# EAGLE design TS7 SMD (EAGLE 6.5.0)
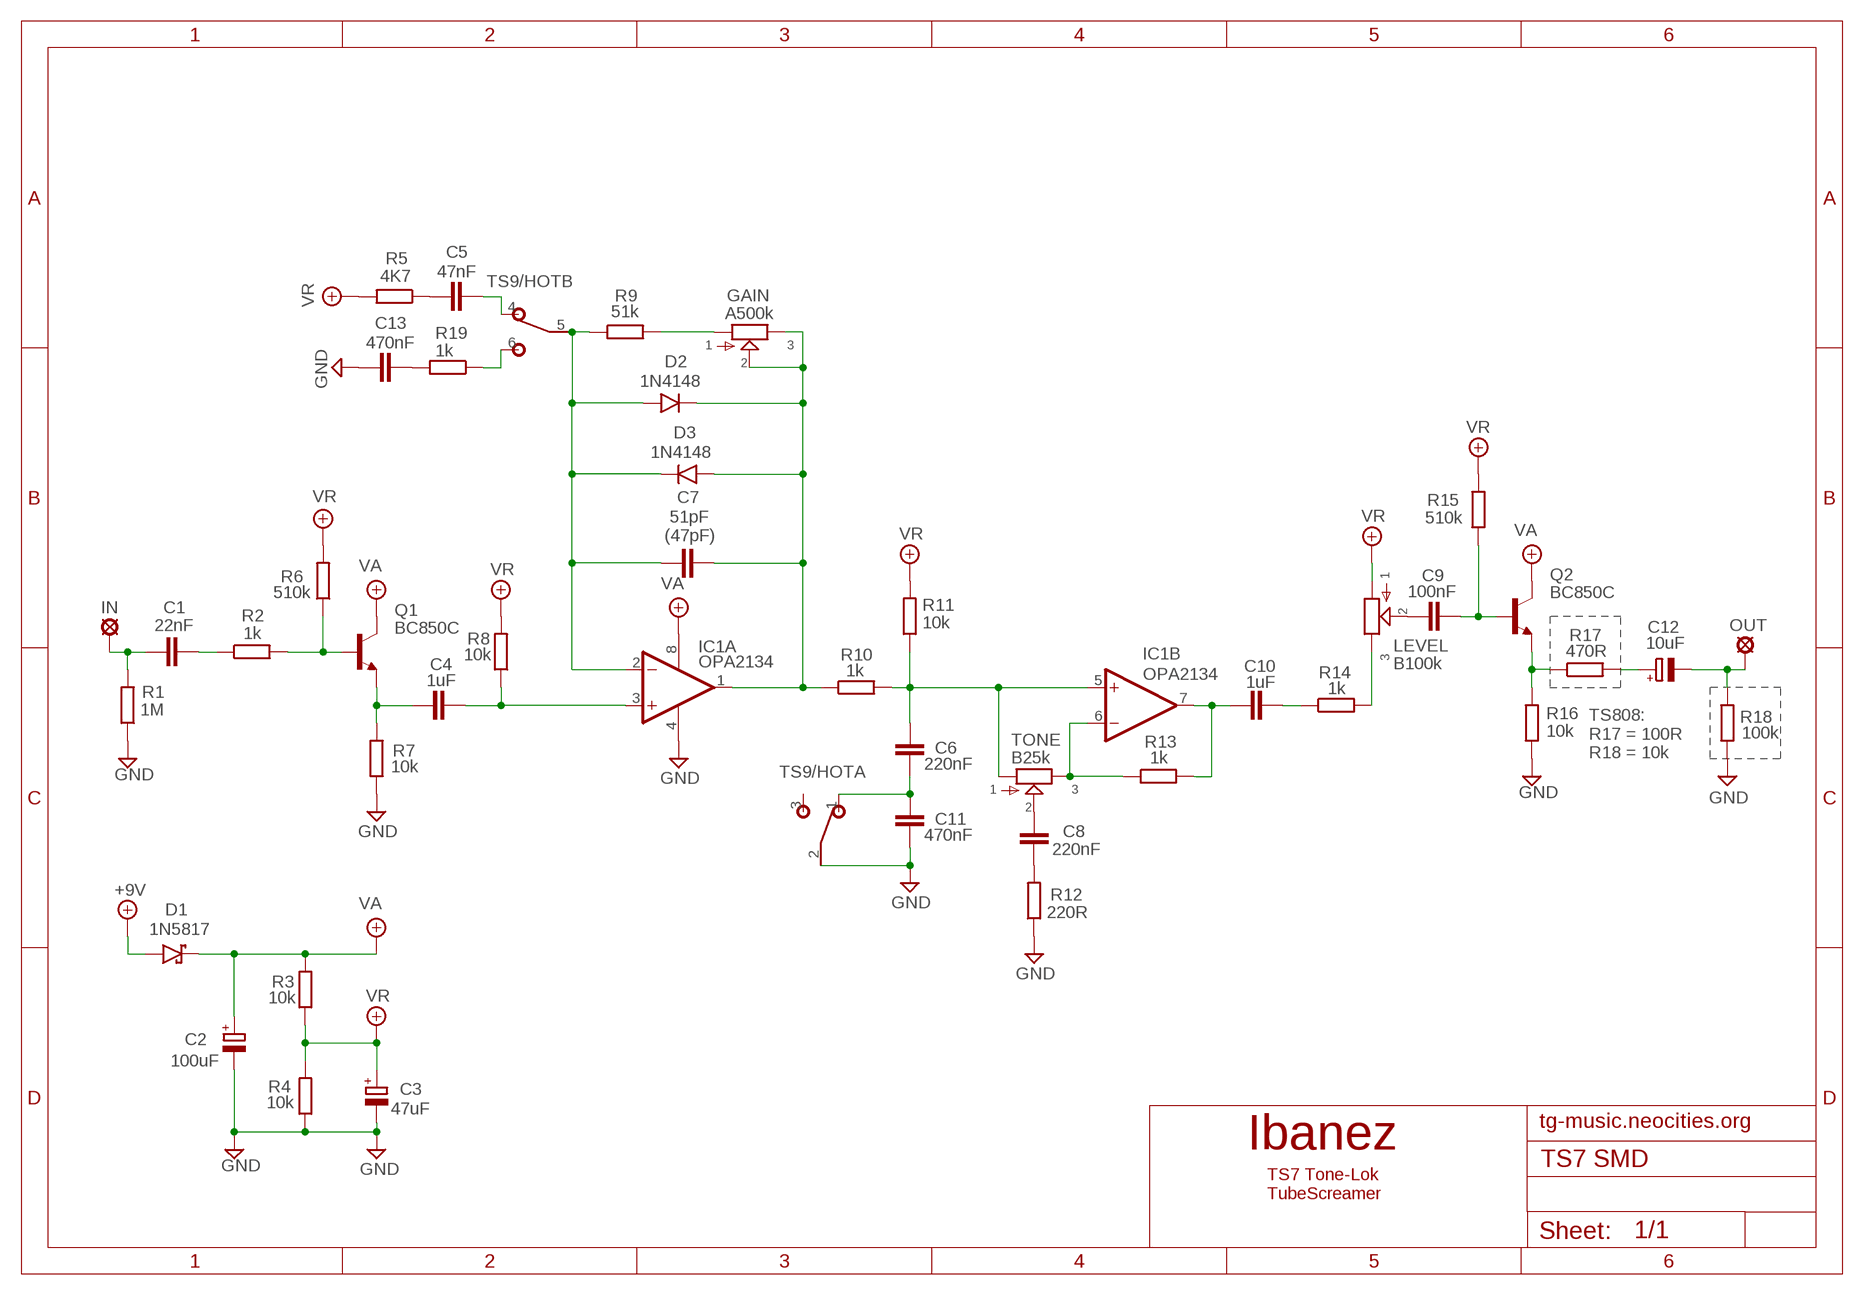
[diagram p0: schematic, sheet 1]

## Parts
+9V  +9V  +9V(T)1  [ROUND]
C1  22nF  C-EUC0805  [C0805]
C2  100uF  CPOL-EUD  [PANASONIC_D]
C3  47uF  CPOL-EUC  [PANASONIC_C]
C4  1uF  C-EUC0805  [C0805]
C5  47nF  C-EUC0805  [C0805]
C6  220nF  C-EUC0805  [C0805]
C7  51pF  C-EUC0805  [C0805]
C8  220nF  C-EUC0805  [C0805]
C9  100nF  C-EUC0805  [C0805]
C10  1uF  C-EUC0805  [C0805]
C11  470nF  C-EUC0805  [C0805]
C12  10uF  CPOL-EUB  [PANASONIC_B]
C13  470nF  C-EUC0805  [C0805]
D1  1N5817  1N5817SMD  [MELF-MLL41_DO213AB]
D2  1N4148  1N4148SMD  [SOD123]
D3  1N4148  1N4148SMD  [SOD123]
GAIN  A500k  POT-EU9MM  [9MM_SNAP-IN_POT]
GND  GND  GND(T)1  [ROUND]
GND1  GND  GND(T)1  [ROUND]
IC1  OPA2134  LM4558D  [SO08]
IN  MCS10B  [MCS10B]
LEVEL  B100k  POT-EU9MM  [9MM_SNAP-IN_POT]
OUT  MCS10B  [MCS10B]
Q1  BC850C  BC847ALT1SMD  [SOT23]
Q2  BC850C  BC847ALT1SMD  [SOT23]
R1  1M  R-EU_R0805  [R0805]
R2  1k  R-EU_R0805  [R0805]
R3  10k  R-EU_R0805  [R0805]
R4  10k  R-EU_R0805  [R0805]
R5  4K7  R-EU_R0805  [R0805]
R6  510k  R-EU_R0805  [R0805]
R7  10k  R-EU_R0805  [R0805]
R8  10k  R-EU_R0805  [R0805]
R9  51k  R-EU_R0805  [R0805]
R10  1k  R-EU_R0805  [R0805]
R11  10k  R-EU_R0805  [R0805]
R12  220R  R-EU_R0805  [R0805]
R13  1k  R-EU_R0805  [R0805]
R14  1k  R-EU_R0805  [R0805]
R15  510k  R-EU_R0805  [R0805]
R16  10k  R-EU_R0805  [R0805]
R17  470R  R-EU_R0805  [R0805]
R18  100k  R-EU_R0805  [R0805]
R19  1k  R-EU_R0805  [R0805]
TONE  B25k  POT-EU9MM  [9MM_SNAP-IN_POT]
TS9/HOT  DPDTTHT  [M9040P2]

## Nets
+9V: +9V.1(+9V) D1.A
GND: C2.- C3.- C11.2 C13.1 GND1.1(GND) GND.1(GND) IC1.4(P:V-) R1.1 R4.1 R7.1 R12.1 R16.1 R18.1 TS9/HOT.2
N$1: C8.1 TONE.2
N$2: C1.2 R2.1
N$3: Q1.1(B) R2.2 R6.1
N$4: C4.2 IC1.3(A:+IN) R8.1
N$5: C7.1 D2.A D3.C IC1.2(A:-IN) R9.1 TS9/HOT.5
N$6: C4.1 Q1.2(E) R7.2
N$7: C8.2 R12.2
N$8: GAIN.1 R9.2
N$9: C9.1 LEVEL.2
N$10: IC1.6(B:-IN) R13.1 TONE.3
N$11: C6.1 IC1.5(B:+IN) R10.2 R11.1 TONE.1
N$12: C6.2 C11.1 TS9/HOT.1
N$13: C7.2 D2.C D3.A GAIN.2 GAIN.3 IC1.1(A:OUT) R10.1
N$15: C10.2 R14.1
N$16: LEVEL.3 R14.2
N$17: Q2.2(E) R16.2 R17.1
N$18: C1.1 IN.MP R1.2
N$19: C9.2 Q2.1(B) R15.1
N$20: C12.+ R17.2
N$21: C12.- OUT.MP R18.2
N$22: C13.2 R19.2
N$23: C5.1 R5.1
N$24: C5.2 TS9/HOT.4
N$25: R19.1 TS9/HOT.6
N$26: C10.1 IC1.7(B:OUT) R13.2
VA: C2.+ D1.C IC1.8(P:V+) Q1.3(C) Q2.3(C) R3.2
VR: C3.+ LEVEL.1 R3.1 R4.2 R5.2 R6.2 R8.2 R11.2 R15.2
Unconnected: TS9/HOT.3

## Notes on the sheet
- (47pF)
- TS808:
  R17 = 100R
  R18 = 10k
- tg-music.neocities.org
- Ibanez
- TS7 Tone-Lok
  TubeScreamer

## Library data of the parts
+9V = gm-supply:+9V(T): +9V Voltage Supply
C1 C4-C11 C13 = rcl:C-EU: CAPACITOR, European symbol
C2 C3 C12 = rcl:CPOL-EU: POLARIZED CAPACITOR, European symbol
D1 = Diodit:1N5817
D2 D3 = Diodit:1N4148: Fast Switching Diode
GAIN LEVEL TONE = potentiometers:POT-EU
GND GND1 = gm-supply:GND(T): Ground
IC1 = Operaatiovahvistimet:*4558: *4558 Op Amp Infamous for its use in tube screamers. This op amp has many manufacturers, hence the leading "*" in the name. The JRC4558 is a widely used example.
IN OUT = Padit:MCS10B: SOLDER PAD
Q1 Q2 = Transistorit:BC847*: NPN Transistor
R1-R19 = rcl:R-EU_: RESISTOR, European symbol
TS9/HOT = Kytkimet:DPDT

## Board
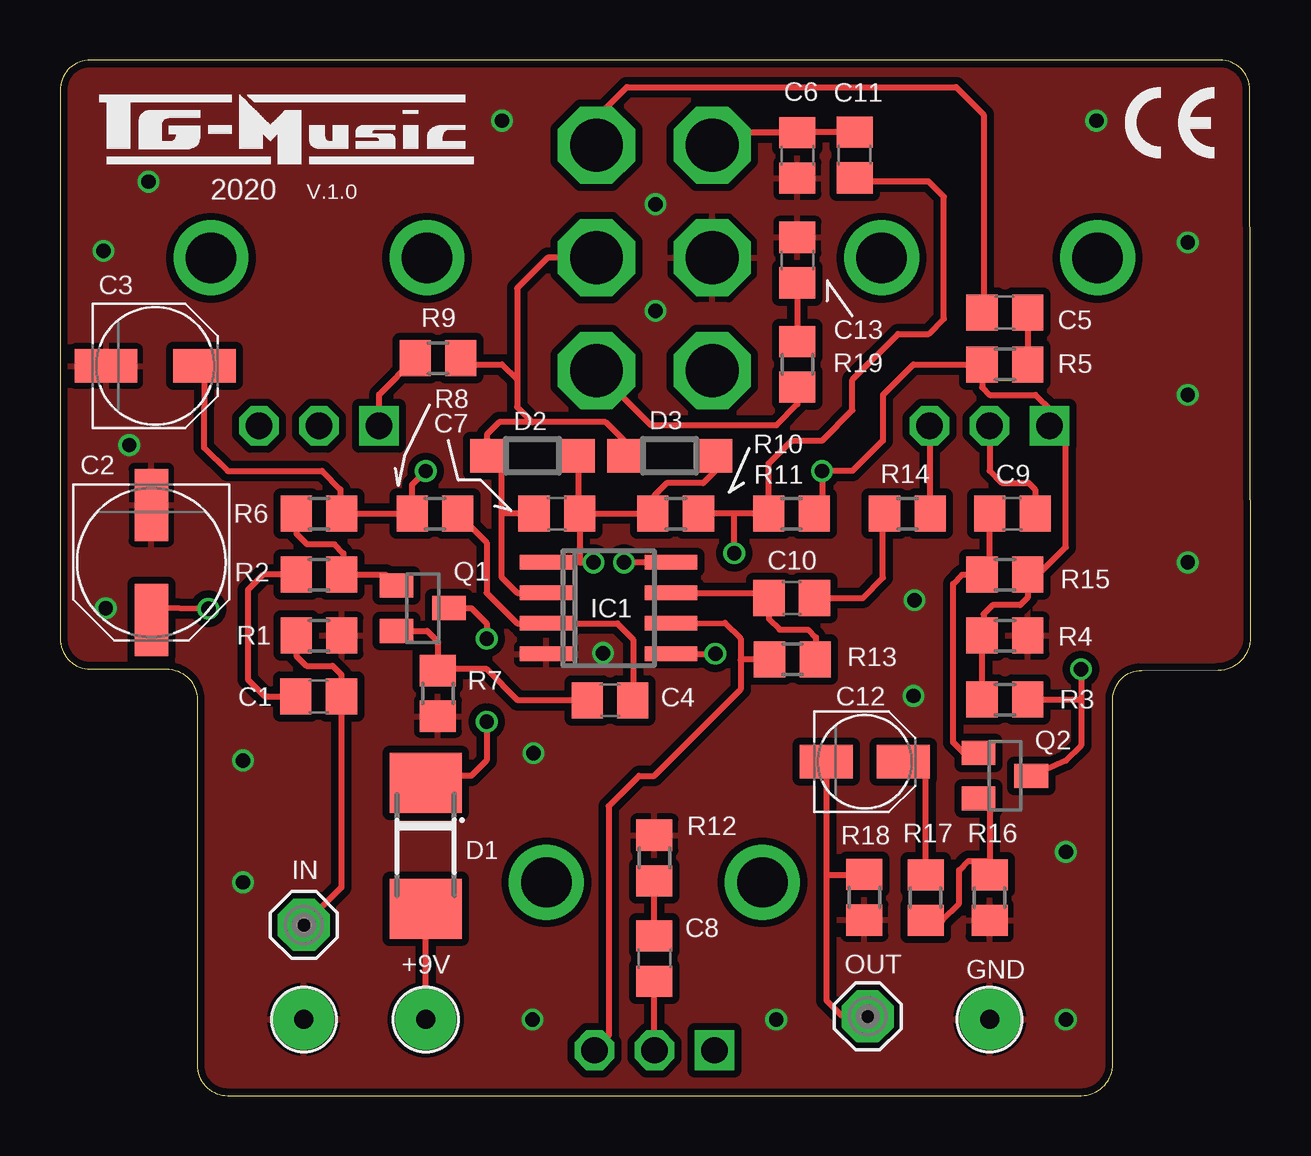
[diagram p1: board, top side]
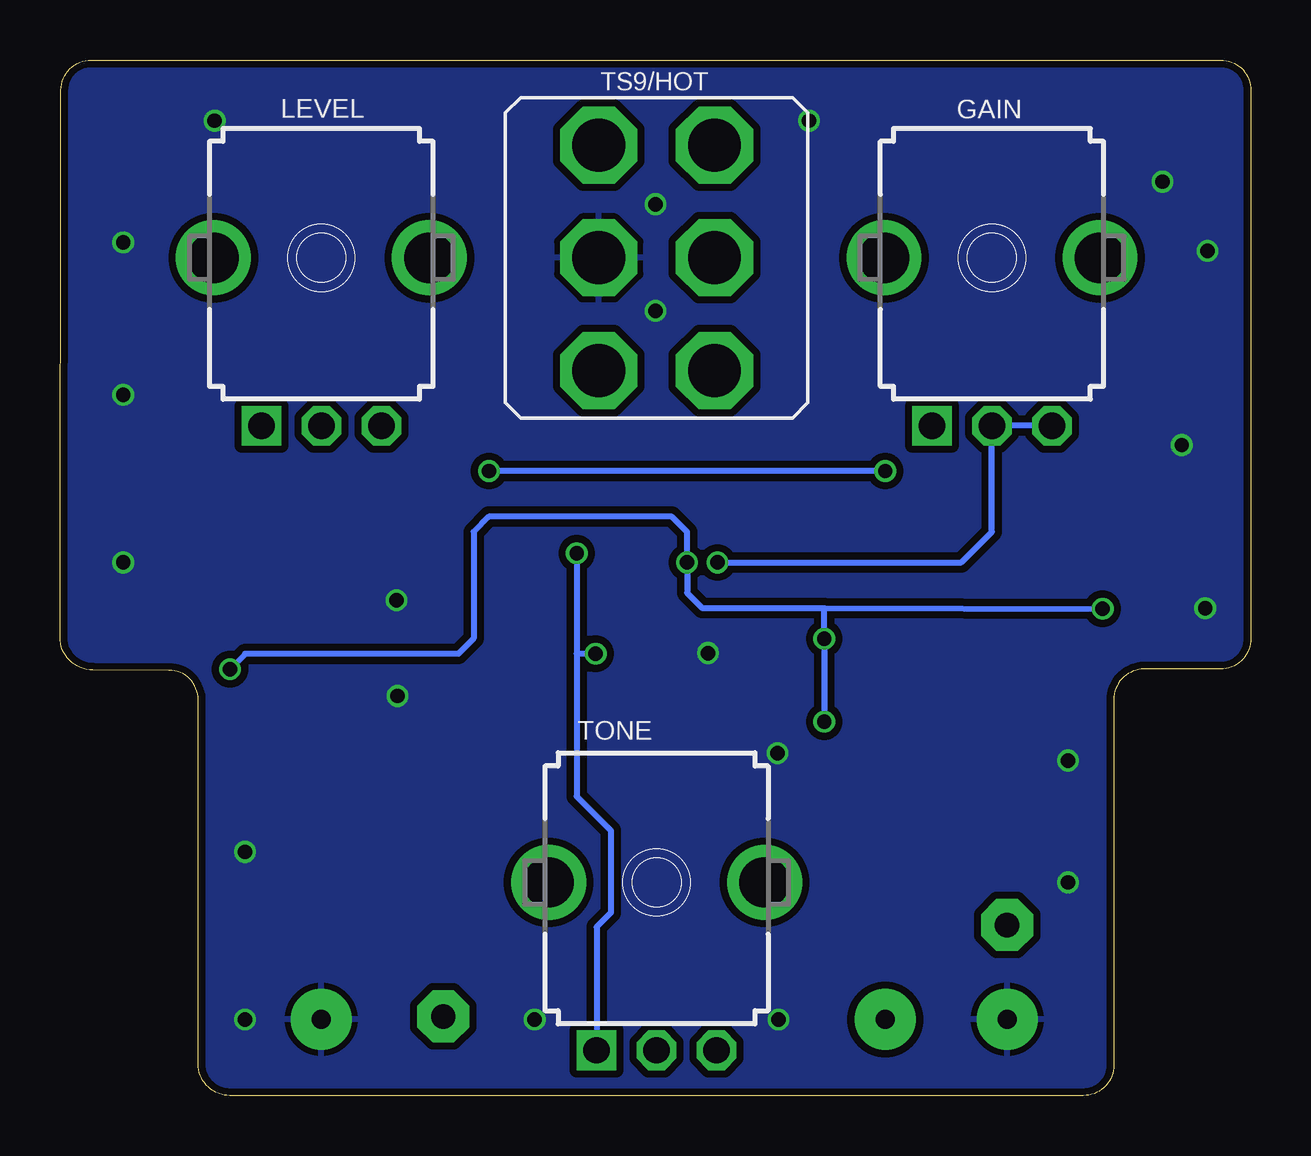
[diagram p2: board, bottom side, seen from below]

Size 49.62 x 43.17 mm. Coordinates in mm from the lower left corner, seen from the top.
Outline: 5.71,16.51 5.71,1.27 arc90 6.99,0 42.55,0 arc90 43.87,1.32 43.87,16.51 arc-90 45.08,17.73 48.26,17.74 arc90 49.62,19.11 49.58,41.91 arc90 48.32,43.17 1.27,43.17 arc90 0,41.9 0,19.05 arc90 1.27,17.78 4.45,17.78 arc-90 5.71,16.51
Copper layers (1*16): Top 0.035mm / dielectric 1.5mm / Bottom 0.035mm
Design rules "ITEADstudio": minimum track width 10mil, minimum drill 12mil, track to track 12mil, track to pad 12mil, pad to pad 12mil, via to via 12mil, smd to smd 0mil, copper to edge 12mil, drill to drill 12mil, minimum pad ring 10mil, minimum via ring 6mil, stop-mask expansion 4mil, vias tented up to drill 100mil, thermal gap 10mil

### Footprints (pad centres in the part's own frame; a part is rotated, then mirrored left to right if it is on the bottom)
ROUND = drill 0.8 pad 2.54: 1 0,0
C0805 = smd 1.3 x 1.5: 1 -0.95,0; 2 0.95,0
PANASONIC_D = smd 3 x 1.4: + 2.4,0; - -2.4,0
PANASONIC_C = smd 2.6 x 1.4: + 2.05,0; - -2.05,0
PANASONIC_B = smd 2.2 x 1.4: + 1.6,0; - -1.6,0
MELF-MLL41_DO213AB = smd 2.5 x 3: A 2.625,0; C -2.625,0
SOD123 = smd 1.4 x 1.4: A 1.9,0; C -1.9,0
9MM_SNAP-IN_POT = drill 1.1 square: 1 -2.5,-7 | drill 1.1 octagon: 2 0,-7; 3 2.5,-7 | drill 2.1 pad 2.794: CHASSIS1 -4.5,0; CHASSIS2 4.5,0
SO08 = smd 0.6 x 2.2: 1 -1.905,-2.6; 2 -0.635,-2.6; 3 0.635,-2.6; 4 1.905,-2.6; 5 1.905,2.6; 6 0.635,2.6; 7 -0.635,2.6; 8 -1.905,2.6
MCS10B = drill 1.016 pad 2.159 octagon: MP 0,0
SOT23 = smd 1 x 1.4: 1 -0.95,-1.1; 2 0.95,-1.1; 3 0,1.1
R0805 = smd 1.3 x 1.5: 1 -0.95,0; 2 0.95,0
M9040P2 = drill 2.2 octagon: 1 -2.413,4.699; 2 -2.413,0; 3 -2.413,-4.699; 4 2.413,4.699; 5 2.413,0; 6 2.413,-4.699

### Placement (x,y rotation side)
+9V  15.24,3.17 0 top
C1  10.78,16.64 180 top
C2  3.81,22.23 270 top
C3  3.97,30.42 0 top
C4  22.92,16.48 0 top
C5  39.37,32.64 180 top
C6  33.11,39.21 90 top
C7  20.7,24.26 0 top
C8  24.77,5.71 90 top
C9  39.68,24.26 180 top
C10  30.49,20.74 0 top
C11  30.72,39.19 270 top
C12  33.53,13.92 0 top
C13  30.72,34.83 270 top
D1  15.24,10.41 270 top
D2  19.68,26.67 180 top
D3  25.4,26.67 0 top
GAIN  10.79,34.92 0 bottom
GND  38.73,3.17 0 top
GND1  10.16,3.17 0 top
IC1  22.86,20.32 270 top
IN  10.16,7.11 0 top
LEVEL  38.73,34.92 0 bottom
OUT  33.66,3.3 0 top
Q1  15.11,20.32 270 top
Q2  39.37,13.34 270 top
R1  10.79,19.18 180 top
R2  10.79,21.72 0 top
R3  39.37,16.51 0 top
R4  39.37,19.18 180 top
R5  39.37,30.48 180 top
R6  10.79,24.26 0 top
R7  15.75,16.76 90 top
R8  15.62,24.26 180 top
R9  15.75,30.73 180 top
R10  25.65,24.26 0 top
R11  30.48,24.26 0 top
R12  24.77,9.91 270 top
R13  30.52,18.19 0 top
R14  35.31,24.26 0 top
R15  39.37,21.72 0 top
R16  38.73,8.26 90 top
R17  36.07,8.26 90 top
R18  33.52,8.27 90 top
R19  30.73,30.48 90 top
TONE  24.77,8.89 0 bottom
TS9/HOT  24.77,34.92 0 bottom

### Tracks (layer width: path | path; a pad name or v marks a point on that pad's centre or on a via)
+9V
  Top 0.254: +9V.1 D1.A
GND  (via drill 0.6)
  other vias: 3.68,38.1 18.41,40.64 43.18,40.64 46.99,35.56 46.99,29.21 46.99,22.23 41.91,10.16 41.91,3.17 29.84,3.17 19.68,3.17 35.56,16.66 7.62,8.89 7.62,13.97 22.63,18.45 19.72,14.28 35.61,20.65 24.81,32.71 24.81,37.16 1.81,35.21 2.88,27.12 1.91,20.32
  pour Top: 5.71,1.27 5.71,16.51 arc90 4.45,17.78 1.27,17.78 arc-90 0,19.05 0,41.91 arc-90 1.27,43.18 48.26,43.18 arc-90 49.53,41.91 49.53,19.05 arc-90 48.26,17.78 45.09,17.78 arc90 43.81,16.51 43.81,1.27 arc-90 42.55,0 6.99,0 arc-90
  pour Bottom: 5.71,1.27 5.71,16.51 arc90 4.45,17.78 1.27,17.78 arc-90 0,19.05 0,41.91 arc-90 1.27,43.18 48.26,43.18 arc-90 49.53,41.91 49.53,19.05 arc-90 48.26,17.78 45.09,17.78 arc90 43.81,16.51 43.81,1.27 arc-90 42.55,0 6.99,0 arc-90
N$1
  Top 0.254: TONE.2 C8.1
N$2
  Top 0.254: R2.1 8.46,21.72 7.83,21.08 7.83,17.35 8.54,16.64 C1.2 | C1.2
N$3
  Top 0.254: Q1.1 13.57,21.72 R2.2 11.81,21.78 11.81,22.61 11.43,22.99 10.29,22.99 9.85,23.43 R6.1
N$4
  Top 0.254: R8.1 17.78,23.05 17.78,20.95 19.05,19.68 IC1.3 23.22,19.68 23.88,19.01 23.88,16.82 C4.2
N$5
  Top 0.254: IC1.2 19.05,20.95 18.41,21.59 18.41,24.26 | D2.A 17.79,26.22 | D2.A 17.79,26.68 | D3.C 23.5,27.3 22.73,28.07 19.68,28.07 | 19.68,28.07 18.29,28.07 17.79,27.56 D2.A | 19.05,29.84 19.05,33.66 20.32,34.92 TS9/HOT.5 | 19.05,29.84 19.05,28.7 19.68,28.07 | R9.1 16.95,30.48 18.41,30.48 19.05,29.84 | 18.41,24.26 18.41,26.04 D2.A | C7.1 18.41,24.26
N$6
  Top 0.254: Q1.2 15.3,19.37 15.75,18.92 R7.2 15.81,17.78 17.78,17.78 19.08,16.48 C4.1
N$7
  Top 0.254: C8.2 R12.2
N$8
  Top 0.254: GAIN.1 13.29,29.23 R9.2
N$9
  Top 0.254: LEVEL.2 38.73,26.05 39.24,25.54 40.35,25.54 40.63,25.27 C9.1
N$10
  Top 0.254: TONE.3 22.86,2.48 22.86,12.06 24.13,13.34 24.77,13.34 28.36,16.93 28.36,18.16 | IC1.6 27.7,19.7 28.36,19.05 28.36,18.16 | R13.1 28.39,18.19 28.36,18.16
N$11  (via drill 0.6)
  Top 0.254: 28.09,24.26 R11.1 29.53,26.36 30.48,27.3 31.75,27.3 33.02,28.57 33.02,29.84 34.92,31.75 36.2,31.75 36.83,32.38 36.83,37.47 36.2,38.1 33.26,38.1 C6.1 | 28.09,24.26 R10.2 26.6,23.82 | v28.09,22.61 28.09,23.71 28.09,24.26 | IC1.5 v27.3,18.41
  Bottom 0.254: v28.09,22.61 28.09,18.41 | 28.09,18.41 28.09,12.47 26.67,11.05 26.67,7.62 27.27,7.03 TONE.1 | v27.3,18.41 28.09,18.41
N$12
  Top 0.254: C6.2 30.72,40.16 C11.1 27.18,40.14 TS9/HOT.1
N$13  (via drill 0.6)
  Top 0.254: IC1.1 v22.23,22.23 21.65,22.23 C7.2 | 21.65,27.24 D2.C 21.59,24.32 C7.2 | C7.2 R10.1 24.77,24.32 24.77,25.02 25.27,25.53 26.8,25.53 27.3,26.03 D3.A
  Bottom 0.254: v22.23,22.23 12.06,22.23 10.79,23.5 GAIN.2 GAIN.3
N$15
  Top 0.254: C10.2 33.44,20.74 34.29,21.59 34.29,24.19 R14.1
N$16
  Top 0.254: LEVEL.3 36.23,25.55 R14.2
N$17
  Top 0.254: Q2.2 38.73,11.92 R16.2 38.67,9.78 37.85,9.78 37.47,9.4 37.47,8 36.77,7.3 R17.1
N$18
  Top 0.254: R1.2 9.85,18.34 10.27,17.92 11.36,17.92 11.72,17.55 C1.1 11.73,8.68 IN.MP
N$19
  Top 0.254: Q2.1 37.66,14.29 37.21,14.73 37.21,21.34 37.59,21.72 R15.1 38.73,21.72 C9.2
N$20
  Top 0.254: R17.2 36.07,13.92 C12.+
N$21
  Top 0.254: R18.2 33.48,9.18 32.01,9.18 31.93,9.1 | C12.- 31.93,9.1 | 31.93,9.1 31.93,3.97 32.55,3.34 33.61,3.34 OUT.MP
N$22
  Top 0.254: C13.2 R19.2
N$23
  Top 0.254: C5.1 R5.1
N$24
  Top 0.254: C5.2 38.48,32.7 38.48,40.89 37.34,42.04 23.62,42.04 22.35,40.77 TS9/HOT.4
N$25
  Top 0.254: R19.1 30.73,28.82 29.84,27.94 24.64,27.94 TS9/HOT.6
N$26
  Top 0.254: IC1.7 29.32,20.95 C10.1 29.54,19.88 29.99,19.43 31.17,19.43 31.5,19.1 31.5,18.22 R13.2
VA  (via drill 0.6)
  Top 0.254: IC1.8 v23.5,22.23 | v42.55,17.78 42.55,16.51 | 42.55,16.51 42.55,14.61 41.91,13.97 Q2.3 | R3.2 42.55,16.51 | v6.18,20.29 3.81,20.32 C2.+ | Q1.3 17.14,20.32 17.78,19.68 v17.78,19.05 | v17.78,15.59 17.78,13.97 17.14,13.34 15.54,13.34 D1.C
  Bottom 0.254: 17.78,20.32 22.86,20.32 23.5,20.95 v23.5,22.23 23.5,23.5 24.13,24.13 31.75,24.13 32.38,23.5 32.38,19.05 33.02,18.41 41.91,18.41 v42.55,17.78 | 17.78,20.32 v6.18,20.29 | 17.78,20.32 v17.78,19.05 v17.78,15.59
VR  (via drill 0.6)
  Top 0.254: v15.24,26.04 14.67,25.47 R8.2 R6.2 11.68,24.32 11.68,25.27 10.92,26.04 6.99,26.04 6,27.01 C3.+ | 31.11,24.45 R11.2 | 31.05,24.13 R11.2 | R3.1 R4.2 38.48,19.24 38.48,20.07 38.86,20.45 40.01,20.45 40.32,20.76 R15.2 40.77,21.72 41.91,22.86 41.91,27.25 LEVEL.1 41.27,27.96 41.27,28.57 40.64,29.21 38.73,29.21 38.42,29.52 R5.2 35.56,30.48 34.29,29.21 34.29,27.3 33.02,26.04 v31.75,26.04 31.75,24.58 R11.2
  Bottom 0.254: v15.24,26.04 v31.75,26.04

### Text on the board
tNames: 2020 | V.1.0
